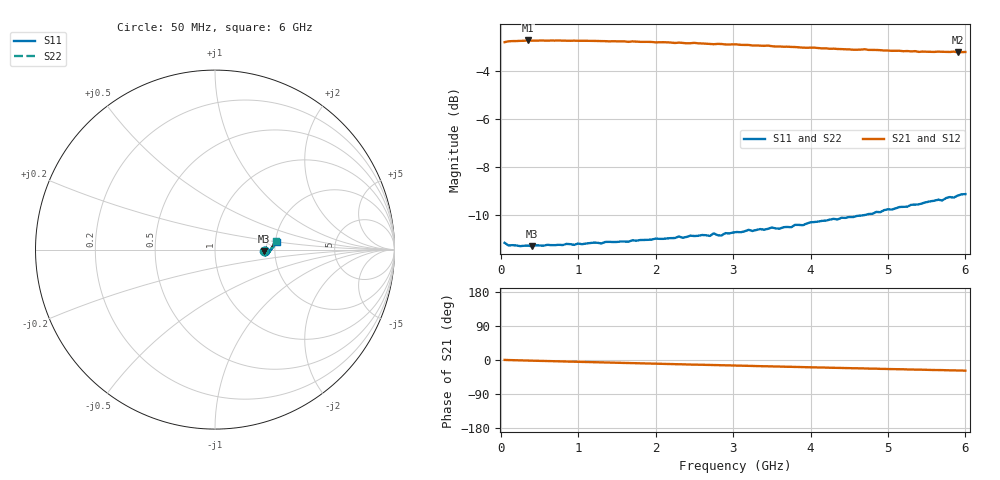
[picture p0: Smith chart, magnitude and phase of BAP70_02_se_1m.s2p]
!	Created	by	janssen	on	Thu	Dec	12	13:21:17	MET	2002
#	HZ	S	MA	R	50
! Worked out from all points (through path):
!   120 points, 50 MHz to 6 GHz, reference 50 ohm
!   highest |S21| = -2.72 dB at 350 MHz (marker M1); lowest = -3.2 dB at 5.9 GHz (marker M2)
!   group delay of S21, straight-line fit = 13.1 ps
!   lowest |S11| = -11.3 dB at 400 MHz (marker M3), VSWR 1.75, Z = 87.3 - j1.73 ohm
!   |S11| at or under -10 dB: start of sweep to 4.713 GHz
!   |S22| runs from -11.3 to -9.2 dB; largest |S21 - S12| = 0.0084
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5e7  0.2764 -1.7  0.7248 0.3  0.7244 0.1  0.2757 -1.5
1e8  0.273 -1.5  0.7278 -0.1  0.727 -0.2  0.2741 -1.4
3.5e8  0.2726 -1.7  0.7308 -1.5  0.7295 -1.5  0.272 -1.8
4e8  0.2719 -1.9  0.7302 -1.7  0.7305 -1.8  0.2719 -2.0
1.05e9  0.2745 -4.2  0.7296 -5.0  0.7292 -4.9  0.2741 -4.3
2.05e9  0.2817 -6.0  0.7244 -10.0  0.7254 -9.9  0.2807 -6.6
2.7e9  0.2857 -6.0  0.7187 -13.0  0.7207 -13.0  0.287 -6.1
2.75e9  0.2892 -5.6  0.7177 -13.3  0.7205 -13.3  0.2879 -6.0
2.85e9  0.2862 -5.5  0.7184 -13.8  0.7197 -13.8  0.289 -5.7
2.9e9  0.2896 -5.5  0.7169 -14.0  0.7212 -14.0  0.29 -5.6
3.05e9  0.2911 -5.6  0.717 -14.8  0.7202 -14.6  0.2899 -5.7
3.2e9  0.2942 -5.0  0.7152 -15.4  0.7176 -15.3  0.2951 -4.7
3.75e9  0.2978 -3.2  0.7084 -18.0  0.7125 -18.1  0.3009 -3.1
4e9  0.305 -2.2  0.7059 -19.3  0.7086 -19.2  0.3026 -1.7
4.05e9  0.3054 -1.6  0.706 -19.4  0.708 -19.4  0.3059 -1.7
4.65e9  0.315 1.1  0.6994 -22.1  0.7041 -22.4  0.3144 1.3
5.05e9  0.3243 2.8  0.6952 -24.0  0.7007 -23.9  0.3257 3.2
5.4e9  0.3325 4.5  0.6917 -25.4  0.6996 -25.6  0.3313 5.0
5.55e9  0.3375 4.9  0.6919 -26.2  0.6987 -26.3  0.3384 5.9
5.7e9  0.3387 5.7  0.6921 -26.7  0.6974 -26.9  0.3408 6.4
5.9e9  0.3468 6.4  0.6904 -27.6  0.6954 -28.0  0.3446 7.2
6e9  0.3493 6.7  0.6914 -28.1  0.6951 -28.4  0.3456 7.7
